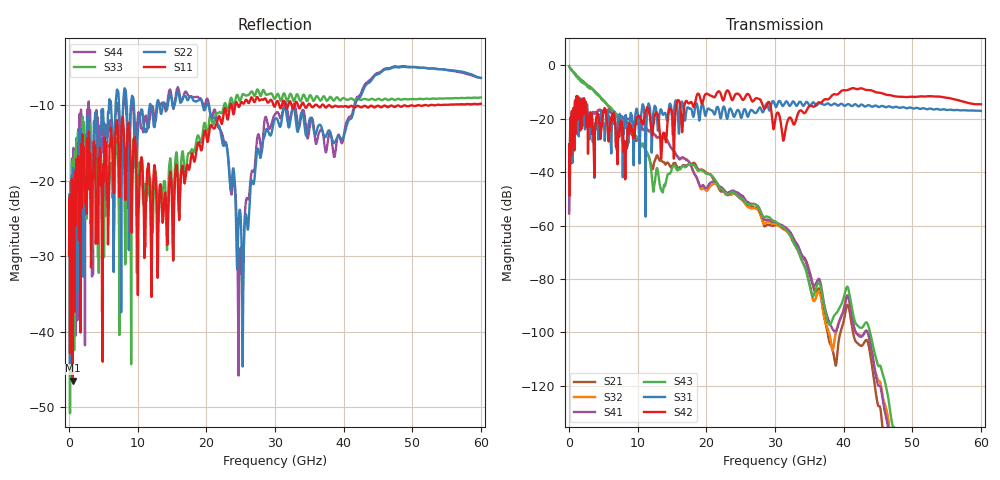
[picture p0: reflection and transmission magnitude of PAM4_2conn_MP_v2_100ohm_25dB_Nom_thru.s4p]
! Info: Touchstone file created by Circ.  Input file=FAB50GbE_2conn_Midplane_Examax_Topo2_v2_100ohm_25dB_Nom.circ
# Hz S RI R 50
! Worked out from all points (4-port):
!   6000 points, 10 MHz to 60 GHz, reference 50 ohm
!   strongest paths, dB at 10 MHz, 15.01 GHz, 30.01 GHz, 45.01 GHz, 60 GHz:
!     S42: -41.7, -18.2, -20.8, -10.2, -14.6
!     S31: -41.7, -19.8, -14.9, -15.5, -17.0
!     S43: -0.3, -38.5, -58.3, -112.3, -172.3
!     S41: -55.4, -31.2, -58.7, -119.7, -179.8
!     S32: -55.4, -31.2, -59.4, -117.8, -176.1
!     S21: -0.3, -37.6, -59.8, -127.2, -186.5
!   lowest |S11| = -46.5 dB at 520 MHz (marker M1), VSWR 1.01, Z = 50.2 + j0.429 ohm
!   |S11| at or under -10 dB: start of sweep to 23.47 GHz; 37.11 GHz to 37.79 GHz (680.3 MHz wide, 1.82 % of centre); 37.96 GHz to 50.77 GHz (12.8 GHz wide, 28.9 % of centre)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
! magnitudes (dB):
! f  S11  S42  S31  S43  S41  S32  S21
! 10 MHz  -29.9  -41.7  -41.7  -0.3  -55.4  -55.4  -0.3
! 520 MHz  -46.5  -29.8  -36.5  -2.1  -24.2  -24.1  -2.1
! 13.89 GHz  -22.3  -25.5  -18.0  -45.0  -27.3  -27.4  -36.4
! 21.29 GHz  -12.9  -11.6  -18.0  -42.8  -43.5  -44.2  -43.7
! 24.87 GHz  -10.0  -11.1  -17.9  -49.6  -48.3  -49.7  -48.3
! 35.06 GHz  -9.8  -15.2  -15.1  -82.6  -78.2  -82.0  -77.4
! 60 GHz  -9.8  -14.6  -17.0  -172.3  -179.8  -176.1  -186.5
